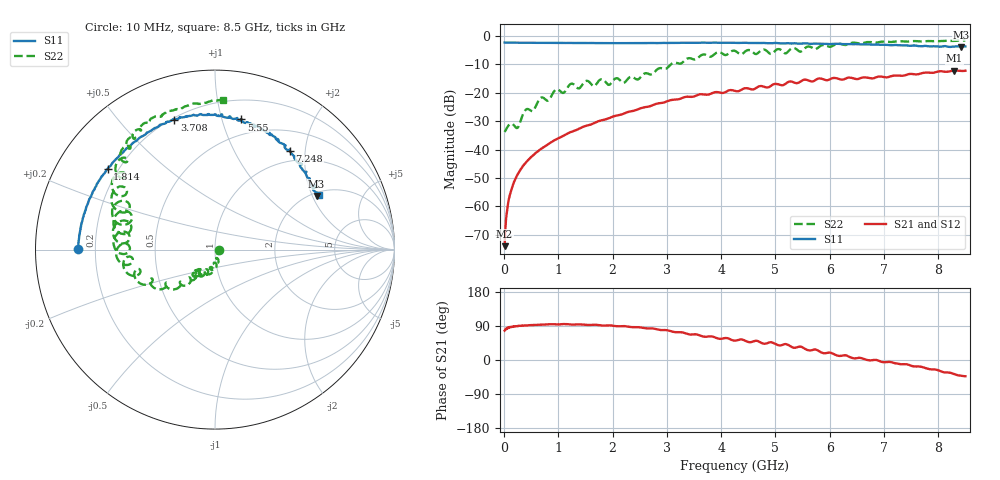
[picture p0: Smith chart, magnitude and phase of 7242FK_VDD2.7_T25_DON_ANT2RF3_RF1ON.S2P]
!Agilent Technologies,E5071C,MY46417908,A.11.23
!Date: Wed Dec 09 15:38:55 2020
!Data & Calibration Information:
!Freq	S11:SOLT2(ON)	S21:SOLT2(ON)	S12:SOLT2(ON)	S22:SOLT2(ON)
!PortZ  Port1:50+j0  Port2:50+j0
!Above PortZ is port z conversion or system Z0 setting when saving the data.
!When reading, reference impedance value at option line is always used.
# Hz S dB R 50
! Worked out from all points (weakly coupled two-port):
!   1601 points, 10 MHz to 8.5 GHz, reference 50 ohm
!   highest |S21| = -12.17 dB at 8.298 GHz (marker M1); lowest = -74.1 dB at 10 MHz (marker M2)
!   lowest |S11| = -3.9 dB at 8.42 GHz (marker M3), VSWR 4.55, Z = 107 + j108 ohm
!   |S11| at or under -10 dB: nowhere
!   |S22| runs from -33.8 to -1.6 dB; largest |S21 - S12| = 0.003
!   S11 on the Smith chart (normalised r, x): 10 MHz: 0.13, +0.00; 1.814 GHz: 0.16, +0.33; 3.708 GHz: 0.21, +0.71; 5.55 GHz: 0.36, +1.16; 7.248 GHz: 0.82, +1.72; 8.5 GHz: 2.13, +2.26
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1e7  -2.32 179.7  -74.05 77.3  -74.39 72.5  -33.80 -0.5
6.836875e7  -2.36 178.5  -59.67 84.8  -59.75 83.9  -31.89 -20.3
1.16125e8  -2.36 177.4  -55.28 86.6  -55.29 87.6  -31.01 -40.6
2.43475e8  -2.38 174.8  -49.00 89.5  -49.02 89.7  -32.42 -59.3
3.28375e8  -2.39 173.0  -46.38 91.0  -46.35 90.9  -28.61 -53.6
9.545125e8  -2.46 160.3  -36.45 94.0  -36.47 94.0  -18.94 -94.7
1.426769e9  -2.47 151.0  -32.27 94.0  -32.27 94.0  -17.61 -106.9
1.814125e9  -2.51 143.1  -29.64 90.9  -29.62 90.9  -15.26 -125.2
2.206788e9  -2.52 135.0  -27.36 89.5  -27.36 89.5  -16.50 -127.2
2.843538e9  -2.51 121.6  -23.73 80.0  -23.74 80.1  -11.49 -131.0
3.708456e9  -2.40 107.4  -20.66 61.3  -20.67 61.3  -6.60 -163.7
4.255e9  -2.42 98.6  -19.35 51.1  -19.36 51.1  -5.26 179.7
4.912975e9  -2.55 88.4  -17.65 47.0  -17.65 46.9  -6.34 165.6
5.045631e9  -2.57 86.9  -16.97 39.3  -16.95 39.3  -4.63 164.7
5.172981e9  -2.60 83.8  -17.00 42.0  -16.98 41.9  -6.08 158.7
5.549725e9  -2.62 78.5  -15.39 29.1  -15.38 29.2  -4.20 157.0
5.671769e9  -2.76 75.7  -16.05 26.0  -15.99 25.9  -4.10 145.7
7.088538e9  -3.17 56.0  -14.44 -5.0  -14.49 -5.0  -2.10 121.7
7.247725e9  -3.23 52.7  -13.93 -9.9  -13.93 -10.0  -1.90 120.6
8.298362e9  -3.73 28.8  -12.17 -37.4  -12.20 -37.3  -1.72 93.9
8.420406e9  -3.88 27.8  -12.32 -41.5  -12.38 -41.7  -1.60 89.8
8.5e9  -3.69 27.7  -12.25 -42.9  -12.32 -42.8  -1.59 87.1
